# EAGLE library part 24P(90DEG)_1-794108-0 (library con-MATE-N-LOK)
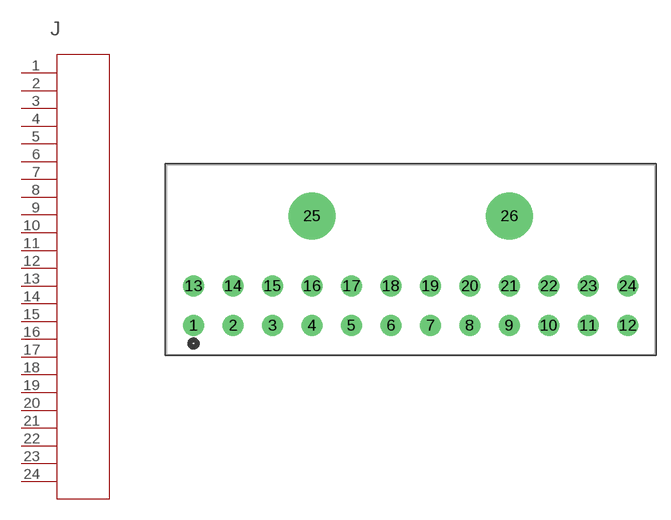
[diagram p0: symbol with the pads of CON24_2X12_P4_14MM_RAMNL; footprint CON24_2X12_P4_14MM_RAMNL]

Designator prefix J

## 24P(90DEG)_1-794108-0 (MANUFACTURER_PART_NUMBER: 17941080; VENDOR: TE Connectivity)  [CON24_2X12_P4_14MM_RAMNL]
1  1  pas
2  2  pas
3  3  pas
4  4  pas
5  5  pas
6  6  pas
7  7  pas
8  8  pas
9  9  pas
10  10  pas
11  11  pas
12  12  pas
13  13  pas
14  14  pas
15  15  pas
16  16  pas
17  17  pas
18  18  pas
19  19  pas
20  20  pas
21  21  pas
22  22  pas
23  23  pas
24  24  pas

## Footprint CON24_2X12_P4_14MM_RAMNL (pad centres in mm)
drill 1.473 pad 1.981: 1 -45.542,-4.14; 2 -41.402,-4.14; 3 -37.262,-4.14; 4 -33.122,-4.14; 5 -28.981,-4.14; 6 -24.841,-4.14; 7 -20.701,-4.14; 8 -16.561,-4.14; 9 -12.421,-4.14; 10 -8.28,-4.14; 11 -4.14,-4.14; 12 0,-4.14; 13 -45.542,0; 14 -41.402,0; 15 -37.262,0; 16 -33.122,0; 17 -28.981,0; 18 -24.841,0; 19 -20.701,0; 20 -16.561,0; 21 -12.421,0; 22 -8.28,0; 23 -4.14,0; 24 0,0
drill 3.912 pad 3.912: 25 -33.122,7.341; 26 -12.421,7.341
